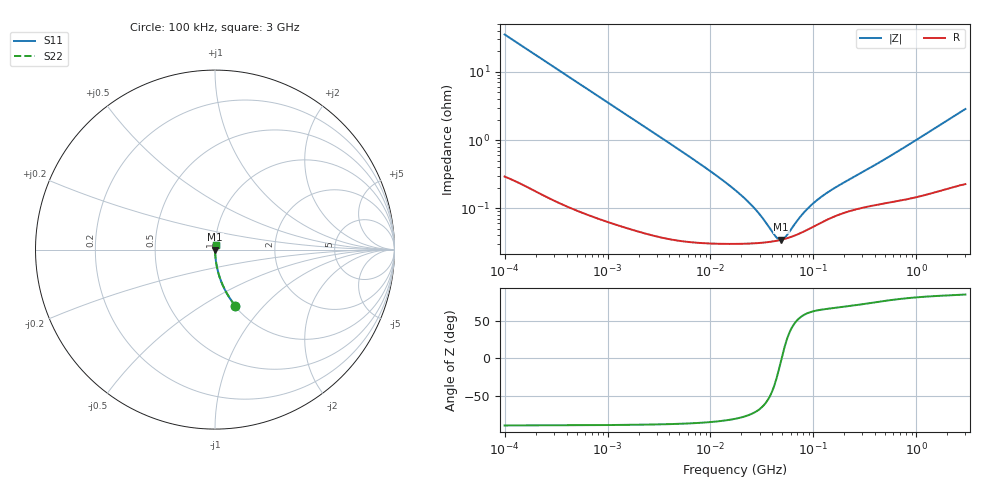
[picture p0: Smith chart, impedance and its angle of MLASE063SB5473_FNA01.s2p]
! MLASE063SB5473_FNA01  S-PARAMETER MODEL  ( Standard Model )
! Model Generated by TAIYO YUDEN Corporation (http://www.ty-top.com)
! Version 1.0
! TAIYO YUDEN Control No. 220601
! Copyright(c) 2013 TAIYO YUDEN CO.,LTD. All Rights Reserved.
! Product Description (link to TY-COMPAS)
! https://ds.yuden.co.jp/TYCOMPAS/or/detail?pn=MLASE063SB5473KFNA01&u=M
! Products Name : Multilayer Ceramic Capacitors
! Characteristics :
!  Capacitance : 0.047 [uF] , Rated Voltage : 16 [V] , TCC : X5R
!  Case Size : 0.6 x 0.3 / 0.024 x 0.012 [mm/inch] , Thickness : 0.3 / 0.012 [mm/inch]
!  (Conditions: Temperature = 25 [degC] , DC Bias Voltage = 0 [V])
! External Node Assignments :
!  1  o---| |---o  2
! GND o---------o GND
! Frequency Range : 100kHz  -  3GHz  [ 401 STEP ]
# MHZ S RI R 50
! Freq[MHz].  S11 Real  S11 Imag  S21 Real  S21 Imag  S12 Real  S12 Imag  S22 Real  S22 Imag
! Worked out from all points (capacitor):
!   401 points, 100 kHz to 3 GHz, reference 50 ohm
!   read as one part in series: C = 45 nF near 105.3 kHz
!   lowest |Z| = 34.5 mohm at 48.56 MHz (marker M1)
!   series resonance near 49.13 MHz, so ESL is about 230 pH
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0.1  0.1129 -0.3124  0.8871 0.3124  0.8871 0.3124  0.1129 -0.3124
0.147195  0.0566 -0.2264  0.9434 0.2264  0.9434 0.2264  0.0566 -0.2264
0.228123  0.0251 -0.1515  0.9749 0.1515  0.9749 0.1515  0.0251 -0.1515
0.344552  0.0117 -0.1019  0.9883 0.1019  0.9883 0.1019  0.0117 -0.1019
0.562235  0.00486 -0.0631  0.9951 0.0631  0.9951 0.0631  0.00486 -0.0631
1.18716  0.00149 -0.0301  0.9985 0.0301  0.9985 0.0301  0.00149 -0.0301
3.161081  0.000508 -0.0114  0.9995 0.0114  0.9995 0.0114  0.000508 -0.0114
9.331111  0.000319 -0.00374  0.9997 0.00374  0.9997 0.00374  0.000319 -0.00374
17.7727  0.000303 -0.00177  0.9997 0.00177  0.9997 0.00177  0.000303 -0.00177
22.99754  0.000304 -0.00123  0.9997 0.00123  0.9997 0.00123  0.000304 -0.00123
28.26337  0.000308 -0.000858  0.9997 0.000858  0.9997 0.000858  0.000308 -0.000858
32.98988  0.000314 -0.000603  0.9997 0.000603  0.9997 0.000603  0.000314 -0.000603
42.68829  0.000331 -0.000207  0.9997 0.000207  0.9997 0.000207  0.000331 -0.000207
46.11977  0.000339 -9.27e-05  0.9997 9.27e-05  0.9997 9.27e-05  0.000339 -9.27e-05
48.55934  0.000345 -1.7e-05  0.9997 1.7e-05  0.9997 1.7e-05  0.000345 -1.7e-05
53.83243  0.000359 0.000134  0.9996 -0.000134  0.9996 -0.000134  0.000359 0.000134
75.25761  0.000434 0.000627  0.9996 -0.000627  0.9996 -0.000627  0.000434 0.000627
97.38194  0.000526 0.00102  0.9995 -0.00102  0.9995 -0.00102  0.000526 0.00102
119.6798  0.000619 0.00134  0.9994 -0.00134  0.9994 -0.00134  0.000619 0.00134
154.8634  0.000744 0.00176  0.9993 -0.00176  0.9993 -0.00176  0.000744 0.00176
547.5153  0.00124 0.0056  0.9988 -0.0056  0.9988 -0.0056  0.00124 0.0056
3000  0.00306 0.0283  0.9969 -0.0283  0.9969 -0.0283  0.00306 0.0283
